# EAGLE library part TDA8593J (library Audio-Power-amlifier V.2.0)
I2C-bus controlled 4 ´ 45 W power amplifier
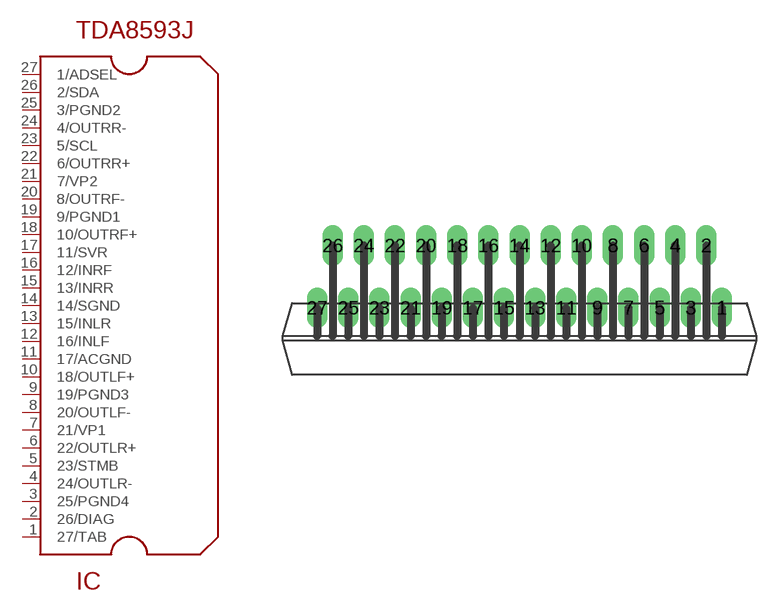
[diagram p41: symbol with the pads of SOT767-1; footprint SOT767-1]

Designator prefix IC

## TDA8593J  [SOT767-1]
1  27/TAB
2  26/DIAG
3  25/PGND4  pwr
4  24/OUTLR-  out
5  23/STMB
6  22/OUTLR+  out
7  21/VP1  pwr
8  20/OUTLF-  out
9  19/PGND3  pwr
10  18/OUTLF+  out
11  17/ACGND  pwr
12  16/INLF  in
13  15/INLR  in
14  14/SGND  pwr
15  13/INRR  in
16  12/INRF  in
17  11/SVR
18  10/OUTRF+  out
19  9/PGND1  pwr
20  8/OUTRF-  out
21  7/VP2  pwr
22  6/OUTRR+  out
23  5/SCL
24  4/OUTRR-  out
25  3/PGND2  pwr
26  2/SDA
27  1/ADSEL

## Footprint SOT767-1 (pad centres in mm)
drill 0.8 long: 1 13,0; 2 12,4; 3 11,0; 4 10,4; 5 9,0; 6 8,4; 7 7,0; 8 6,4; 9 5,0; 10 4,4; 11 3,0; 12 2,4; 13 1,0; 14 0,4; 15 -1,0; 16 -2,4; 17 -3,0; 18 -4,4; 19 -5,0; 20 -6,4; 21 -7,0; 22 -8,4; 23 -9,0; 24 -10,4; 25 -11,0; 26 -12,4; 27 -13,0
